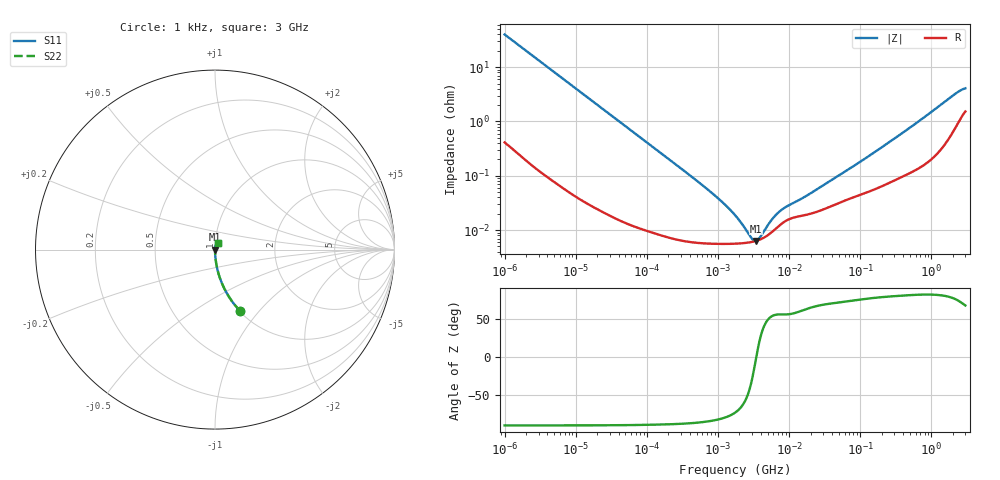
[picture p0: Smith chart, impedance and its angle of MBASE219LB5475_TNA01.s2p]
! MBASE219LB5475_TNA01  S-PARAMETER MODEL  ( Standard Model )
! Model Generated by TAIYO YUDEN Corporation (http://www.ty-top.com)
! Version 1.0
! TAIYO YUDEN Control No. 220601
! Copyright(c) 2012 TAIYO YUDEN CO.,LTD. All Rights Reserved.
! Product Description (link to TY-COMPAS)
! https://ds.yuden.co.jp/TYCOMPAS/or/detail?pn=MBASE219LB5475KTNA01&u=M
! Products Name : Multilayer Ceramic Capacitors
! Characteristics :
!  Capacitance : 4.7 [uF] , Rated Voltage : 16 [V] , TCC : X5R
!  Case Size : 2.0 x 1.25 / 0.079 x 0.049 [mm/inch] , Thickness : 0.85 / 0.033 [mm/inch]
!  (Conditions: Temperature = 25 [degC] , DC Bias Voltage = 0 [V])
! External Node Assignments :
!  1  o---| |---o  2
! GND o---------o GND
! Frequency Range : 1kHz  -  3GHz  [ 401 STEP ]
# MHZ S RI R 50
! Freq[MHz].  S11 Real  S11 Imag  S21 Real  S21 Imag  S12 Real  S12 Imag  S22 Real  S22 Imag
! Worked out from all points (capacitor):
!   401 points, 1 kHz to 3 GHz, reference 50 ohm
!   read as one part in series: C = 3.97 uF near 1.077 kHz
!   lowest |Z| = 6.32 mohm at 3.389 MHz (marker M1)
!   series resonance near 3.446 MHz, so ESL is about 540 pH
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0.001  0.1407 -0.3426  0.8593 0.3426  0.8593 0.3426  0.1407 -0.3426
0.001685  0.0557 -0.2246  0.9443 0.2246  0.9443 0.2246  0.0557 -0.2246
0.00306  0.0182 -0.1292  0.9818 0.1292  0.9818 0.1292  0.0182 -0.1292
0.005768  0.00555 -0.0697  0.9944 0.0697  0.9944 0.0697  0.00555 -0.0697
0.01216  0.00146 -0.0333  0.9985 0.0333  0.9985 0.0333  0.00146 -0.0333
0.147855  8.99e-05 -0.00279  0.9999 0.00279  0.9999 0.00279  8.99e-05 -0.00279
0.791611  5.64e-05 -0.000499  0.9999 0.000499  0.9999 0.000499  5.64e-05 -0.000499
1.238299  5.58e-05 -0.000294  0.9999 0.000294  0.9999 0.000294  5.58e-05 -0.000294
1.732051  5.62e-05 -0.000181  0.9999 0.000181  0.9999 0.000181  5.62e-05 -0.000181
2.514714  5.84e-05 -7.84e-05  0.9999 7.84e-05  0.9999 7.84e-05  5.84e-05 -7.84e-05
3.388684  6.3e-05 -4.08e-06  0.9999 4.08e-06  0.9999 4.08e-06  6.3e-05 -4.08e-06
4.399271  7.24e-05 6.07e-05  0.9999 -6.07e-05  0.9999 -6.07e-05  7.24e-05 6.07e-05
4.739869  7.67e-05 7.95e-05  0.9999 -7.95e-05  0.9999 -7.95e-05  7.67e-05 7.95e-05
6.153411  0.0001 0.000145  0.9999 -0.000145  0.9999 -0.000145  0.0001 0.000145
7.696136  0.000129 0.000194  0.9999 -0.000194  0.9999 -0.000194  0.000129 0.000194
21.06097  0.000204 0.000453  0.9998 -0.000453  0.9998 -0.000453  0.000204 0.000453
93.58162  0.000435 0.00166  0.9996 -0.00166  0.9996 -0.00166  0.000435 0.00166
256.0921  0.000758 0.00411  0.9992 -0.00411  0.9992 -0.00411  0.000758 0.00411
650.4536  0.00145 0.00979  0.9986 -0.00979  0.9986 -0.00979  0.00145 0.00979
2144.796  0.00835 0.0308  0.9917 -0.0308  0.9917 -0.0308  0.00835 0.0308
2584.342  0.0126 0.035  0.9874 -0.035  0.9874 -0.035  0.0126 0.035
3000  0.0164 0.0367  0.9836 -0.0367  0.9836 -0.0367  0.0164 0.0367
